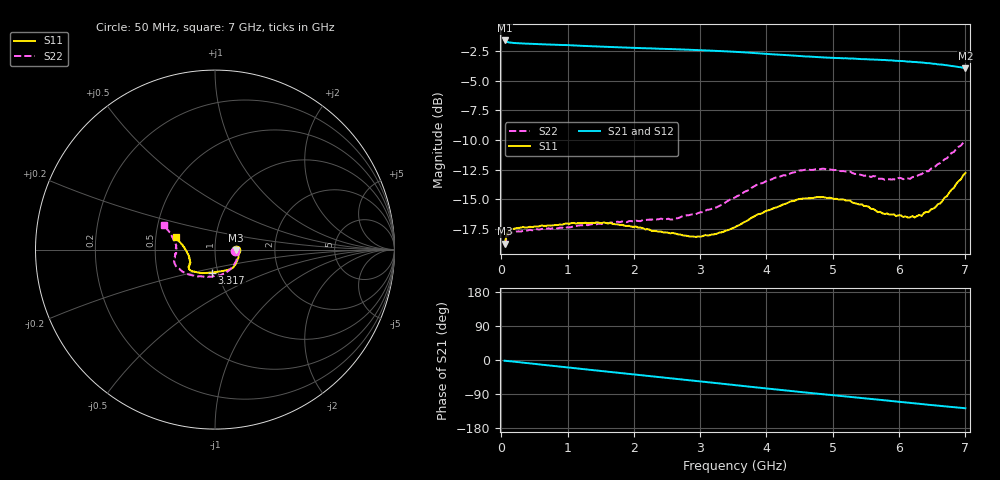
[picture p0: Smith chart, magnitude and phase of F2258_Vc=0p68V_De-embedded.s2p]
! Integrated Device Technology
! Corporate Headquarters
! 6024 Silver Creek Valley Road
! San Jose, CA 95138  USA
! Phone:  1-408-284-8200
! Toll Free:  1-800-223-1366
! Webpage:  http://www.idt.com/
! Timing and RF Division
! 515 Groton Road, Suite 102
! Westford, MA 01886-6024
! Device:  F2258
! Description: Voltage Variable RF Attenuator
! Frequency:  50.0 -  6000.00 MHz
! Package:  3x3 mm Thin QFN Plastic Package: 16 pin
! Ports:  2 RF, 2 DC
!  Pin  1  = NC
!  Pin  2  = NC
!  Pin  3  = RF2  = Port 2
!  Pin  4  = GND
!  Pin  5  = Vdd
!  Pin  6  = NC
!  Pin  7  = VCTRL
!  Pin  8  = NC
!  Pin  9  = GND
!  Pin 10  = RF1  = Port 1
!  Pin 11  = NC
!  Pin 12  = NC
!  Pin 13  = NC
!  Pin 14  = NC
!  Pin 15  = NC
!  Pin 16  = NC
! Vcntrl:  0.680 Volts
! Vdd:  +3.300 Volts
! Current:  1.117 mA
! Data:  The device was measured on a the F2258 evaluation board which has
!  individual transmission lines to the RF pins.  Data was collected
!  using a calibrated network analyzer.  The evaluation board was
!  de-embedded using a TRL calibration technique.
!  The reference plane is the edge of the package pin.
! Misc:  SN 10
!  Action Tracker AT0285
! Date Measured:  2014-12-10
! Date:  2016-01-13  MJV
! Note:
!  Integrated Device Technology supplies this data as a sample of measured
!  data at the package pin for this product.  Your particular data for this
!  product may vary.
!  Data was taken at 25 degrees C.
!  Integrated Device Technology reserves the right to change this data at anytime.
!Freq_(GHz)  S11M_(dB)  S11P_(deg)  S21M_(dB)  S21P_(deg)  S12M_(dB)  S12P_(deg)  S22M_(dB)  S22P_(deg)
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# GHz S dB R 50
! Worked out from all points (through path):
!   201 points, 50 MHz to 7 GHz, reference 50 ohm
!   highest |S21| = -1.62 dB at 50 MHz (marker M1); lowest = -4.0 dB at 7 GHz (marker M2)
!   group delay of S21, straight-line fit = 50.4 ps
!   lowest |S11| = -18.7 dB at 50 MHz (marker M3), VSWR 1.26, Z = 63 - j0.505 ohm
!   |S11| at or under -10 dB: start of sweep to end of sweep
!   |S22| runs from -19.0 to -10.1 dB; largest |S21 - S12| = 0.0011
!   S11 on the Smith chart (normalised r, x): 50 MHz: 1.26, -0.01; 3.317 GHz: 0.94, -0.24; 7 GHz: 0.64, +0.09
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0.05  -18.75 -2.0  -1.62 -2.0  -1.62 -2.0  -18.96 -2.7
0.08475  -17.90 -3.3  -1.74 -2.5  -1.74 -2.5  -18.16 -4.1
0.15425  -17.51 -5.3  -1.82 -3.7  -1.81 -3.7  -17.83 -7.1
0.71025  -17.21 -23.4  -1.96 -14.2  -1.96 -14.2  -17.46 -29.8
0.9535  -17.07 -31.9  -2.01 -18.8  -2.01 -18.8  -17.49 -40.6
1.2315  -17.03 -39.0  -2.08 -23.9  -2.08 -23.9  -17.20 -50.6
1.6485  -17.01 -48.1  -2.17 -31.5  -2.18 -31.5  -16.97 -63.5
2.37825  -17.74 -62.7  -2.32 -44.8  -2.31 -44.8  -16.69 -83.1
2.58675  -17.84 -68.3  -2.35 -48.7  -2.35 -48.7  -16.70 -89.7
2.93425  -18.17 -80.6  -2.43 -55.1  -2.42 -55.1  -16.27 -102.1
3.3165  -17.80 -97.5  -2.52 -62.3  -2.51 -62.3  -15.49 -117.5
3.525  -17.36 -107.4  -2.58 -66.3  -2.57 -66.3  -14.86 -125.7
4.0115  -15.95 -126.5  -2.76 -75.3  -2.75 -75.3  -13.42 -142.6
4.46325  -15.03 -137.8  -2.92 -83.5  -2.92 -83.5  -12.63 -154.7
4.7065  -14.90 -141.2  -3.00 -87.8  -3.00 -87.8  -12.52 -159.4
5.2625  -15.12 -147.3  -3.15 -97.4  -3.16 -97.4  -12.67 -168.4
5.85325  -16.30 -155.1  -3.30 -107.6  -3.30 -107.6  -13.33 -179.4
6.166  -16.53 -163.2  -3.40 -113.2  -3.40 -113.2  -13.29 173.9
6.2355  -16.54 -166.8  -3.44 -114.3  -3.43 -114.4  -13.10 171.8
6.444  -16.09 -175.7  -3.53 -118.1  -3.54 -118.1  -12.65 167.0
6.722  -14.75 171.7  -3.71 -122.9  -3.71 -122.9  -11.56 159.5
7  -12.79 162.3  -3.95 -127.4  -3.96 -127.4  -10.06 154.1
